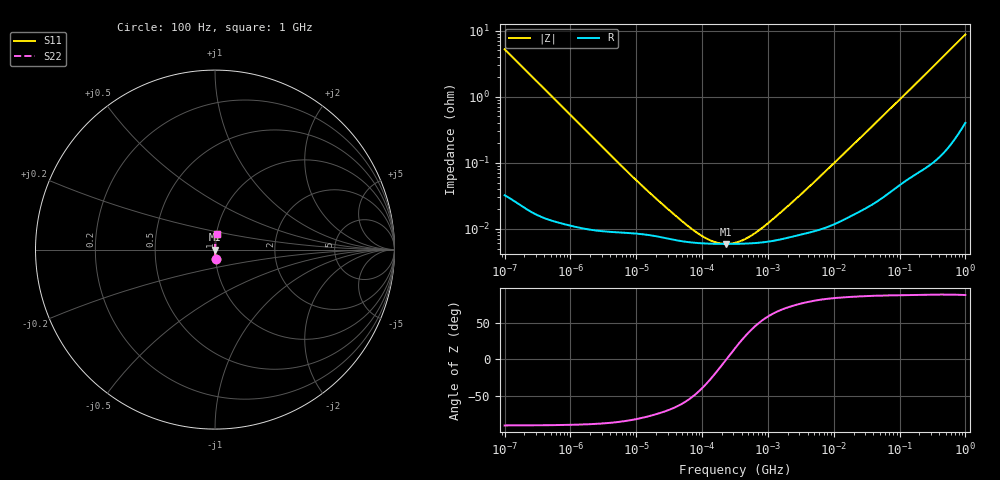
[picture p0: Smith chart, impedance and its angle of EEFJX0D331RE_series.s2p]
!  *** S-Parameter ***
!  Copyright (C) Panasonic Industry Corporation
!  Conductive Polymer Aluminum Electrolytic Capacitor (SP-Cap)
!  Parts No. EEFJX0D331RE
!  Connection Mode : Series
!  1  o---||---o  2
!  GND o--------o GND
!  Conditions : Temperature = 20   DC Bias = 0 V
! Frequency Range : 100Hz  -  1GHz  [ 401 Steps ]
# Hz S RI R 50
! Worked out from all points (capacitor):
!   401 points, 100 Hz to 1 GHz, reference 50 ohm
!   read as one part in series: C = 306 uF near 108.4 Hz
!   lowest |Z| = 5.88 mohm at 229.1 kHz (marker M1)
!   series resonance near 233.3 kHz, so ESL is about 1.5 nH
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100  0.00301 -0.0518  0.997 0.0518  0.997 0.0518  0.00301 -0.0518
108.3927  0.0026 -0.0479  0.9974 0.0479  0.9974 0.0479  0.0026 -0.0479
296.8247  0.000474 -0.0176  0.9995 0.0176  0.9995 0.0176  0.000474 -0.0176
1487.647  0.000114 -0.00353  0.9999 0.00353  0.9999 0.00353  0.000114 -0.00353
8081.649  8.61e-05 -0.000658  0.9999 0.000658  0.9999 0.000658  8.61e-05 -0.000658
22130.95  7.55e-05 -0.00025  0.9999 0.00025  0.9999 0.00025  7.55e-05 -0.00025
49545.02  6.46e-05 -0.000113  0.9999 0.000113  0.9999 0.000113  6.46e-05 -0.000113
63095.73  6.25e-05 -8.68e-05  0.9999 8.68e-05  0.9999 8.68e-05  6.25e-05 -8.68e-05
68391.16  6.19e-05 -7.92e-05  0.9999 7.92e-05  0.9999 7.92e-05  6.19e-05 -7.92e-05
77179.15  6.12e-05 -6.86e-05  0.9999 6.86e-05  0.9999 6.86e-05  6.12e-05 -6.86e-05
229086.8  5.88e-05 -9.2e-07  0.9999 9.2e-07  0.9999 9.2e-07  5.88e-05 -9.2e-07
316227.8  5.89e-05 1.59e-05  0.9999 -1.59e-05  0.9999 -1.59e-05  5.89e-05 1.59e-05
737055.2  6.13e-05 7.25e-05  0.9999 -7.25e-05  0.9999 -7.25e-05  6.13e-05 7.25e-05
831763.8  6.21e-05 8.36e-05  0.9999 -8.36e-05  0.9999 -8.36e-05  6.21e-05 8.36e-05
1059254  6.41e-05 0.000109  0.9999 -0.000109  0.9999 -0.000109  6.41e-05 0.000109
1650061  6.97e-05 0.000171  0.9999 -0.000171  0.9999 -0.000171  6.97e-05 0.000171
4704354  8.99e-05 0.000467  0.9999 -0.000467  0.9999 -0.000467  8.99e-05 0.000467
6.99842e7  0.000389 0.00635  0.9996 -0.00635  0.9996 -0.00635  0.000389 0.00635
3.368992e8  0.0019 0.0294  0.9981 -0.0294  0.9981 -0.0294  0.0019 0.0294
5.688529e8  0.0042 0.0493  0.9958 -0.0493  0.9958 -0.0493  0.0042 0.0493
9.225714e8  0.00984 0.0792  0.9902 -0.0792  0.9902 -0.0792  0.00984 0.0792
1e9  0.0114 0.0857  0.9886 -0.0857  0.9886 -0.0857  0.0114 0.0857
